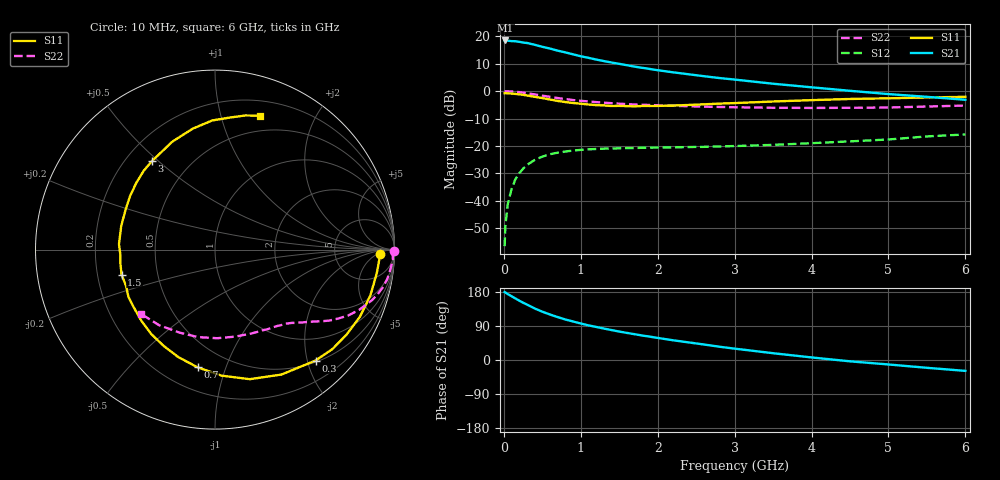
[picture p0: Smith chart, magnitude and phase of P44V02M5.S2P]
! SIEMENS Small Signal Semiconductors
! BFP182
! Si NPN RF Bipolar Junction Transistor in SOT143
! VCE = 4 V  IC = 2.5 mA
! Common Emitter S-Parameters:  March  1996
# GHz  S  MA  R  50
!  f  S11  S21  S12  S22
! GHz  MAG  ANG  MAG  ANG  MAG  ANG  MAG  ANG
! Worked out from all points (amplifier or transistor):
!   36 points, 10 MHz to 6 GHz, reference 50 ohm
!   highest |S21| = 18.5 dB at 20 MHz (marker M1)
!   |S21| within 3 dB of that: start of sweep to 606.4 MHz
!   unconditionally stable (mu >= 1): 2.062 GHz to 5.892 GHz
!   at 250 MHz: K = 0.14, MSG = 23.0 dB, |S12| = -28.3 dB
!   at 1.4 GHz: K = 0.73, MSG = 15.7 dB, |S12| = -20.9 dB
!   at 6 GHz: K = 0.98, MSG = 6.3 dB, |S12| = -15.8 dB
!   S11 on the Smith chart (normalised r, x): 10 MHz: 21, -7; 300 MHz: 0.53, -2.15; 700 MHz: 0.34, -0.80; 1.5 GHz: 0.30, -0.12; 3 GHz: 0.31, +0.48; 6 GHz: 0.34, +1.34
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0.01  0.9177 -1.7  8.218 179.0  0.0015 81.5  0.9947 -0.6
0.02  0.9175 -3.3  8.371 178.1  0.0035 87.0  0.99 -1.3
0.05  0.911 -8.2  8.319 174.1  0.0086 88.6  0.9928 -3.2
0.15  0.8901 -24.8  8.108 162.4  0.0248 75.8  0.974 -9.7
0.2  0.8732 -32.7  7.917 156.7  0.0318 71.4  0.9583 -12.7
0.3  0.8343 -47.8  7.534 146.4  0.0451 63.3  0.9174 -18.0
0.4  0.7885 -62.0  6.995 136.1  0.0556 56.2  0.8714 -22.6
0.5  0.7474 -75.0  6.412 127.5  0.0641 49.5  0.8281 -26.3
0.6  0.703 -87.1  5.96 120.0  0.071 44.7  0.7869 -29.2
0.7  0.663 -98.4  5.453 113.2  0.0756 40.2  0.7487 -31.9
0.8  0.6328 -108.9  5.076 106.9  0.0794 36.5  0.7158 -33.9
0.9  0.6076 -118.2  4.673 101.6  0.0828 33.5  0.6876 -35.6
1.1  0.5707 -136.0  4.041 91.4  0.087 28.7  0.6471 -38.6
1.3  0.5498 -151.1  3.526 83.0  0.0896 24.9  0.6157 -41.3
1.5  0.539 -165.0  3.141 75.0  0.0908 22.7  0.5901 -43.8
1.8  0.536 176.8  2.658 64.6  0.093 20.4  0.5647 -47.5
2.2  0.5451 156.5  2.201 52.0  0.0944 19.0  0.5398 -53.4
3  0.6055 125.5  1.624 30.0  0.0999 18.9  0.5084 -67.2
3.5  0.647 111.5  1.363 17.9  0.105 19.2  0.4974 -77.2
4.5  0.7198 91.2  1.014 -3.5  0.1216 19.6  0.4967 -101.0
5.5  0.7665 77.2  0.787 -20.6  0.1497 18.3  0.524 -126.6
6  0.7871 71.4  0.696 -28.7  0.1625 15.1  0.5464 -139.2
